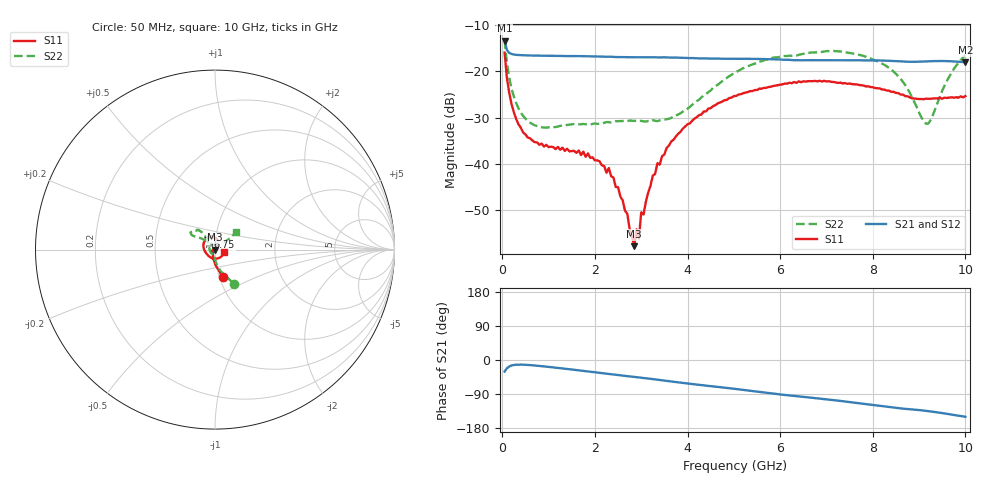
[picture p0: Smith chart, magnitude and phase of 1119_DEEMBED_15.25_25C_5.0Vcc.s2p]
!Hittite Microwave Corp.
!Digital Attenuator/PhaseShifter Rev 1.4.0
!Filename: C:\DATA\DATA\1119_DEEMBED_15.25_25C_5.0Vcc.s2p
!VNA ID: Agilent Technologies,N5224A,MY51441122,A.10.45.03
!Device type:
!2 Port Calibration.
!Temp(C): 25
!Lot Number:
!Serial Number:
!Operator:
!Misc:
!Attenuator:  15.250
# GHZ S DB R 50.0
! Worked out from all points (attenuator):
!   200 points, 50 MHz to 10 GHz, reference 50 ohm
!   highest |S21| = -13.29 dB at 50 MHz (marker M1); lowest = -18.0 dB at 10 GHz (marker M2)
!   lowest |S11| = -57.9 dB at 2.85 GHz (marker M3), VSWR 1.00, Z = 50 - j0.128 ohm
!   |S11| at or under -10 dB: start of sweep to end of sweep
!   |S22| runs from -32.2 to -13.3 dB; largest |S21 - S12| = 0.00049
!   S11 on the Smith chart (normalised r, x): 50 MHz: 1.04, -0.33; 6.75 GHz: 0.92, +0.13; 10 GHz: 1.11, -0.03
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0.05  -15.92 -74.2  -13.29 -30.4  -13.30 -30.5  -13.28 -61.1
0.1  -21.43 -88.5  -15.38 -21.8  -15.38 -21.8  -18.20 -75.7
0.2  -27.09 -102.7  -16.21 -14.5  -16.22 -14.5  -23.71 -87.1
0.45  -33.23 -125.1  -16.49 -12.3  -16.50 -12.4  -29.63 -97.7
0.85  -35.65 -147.3  -16.58 -16.2  -16.58 -16.2  -32.10 -106.0
1.75  -37.39 -159.4  -16.69 -28.8  -16.69 -28.8  -31.39 -116.4
2.3  -40.94 -162.7  -16.80 -37.0  -16.80 -37.0  -31.00 -131.7
2.7  -50.87 -115.3  -16.91 -42.6  -16.92 -42.7  -30.76 -142.3
2.85  -57.88 -89.0  -16.92 -44.8  -16.93 -44.8  -30.74 -148.8
2.9  -54.24 -22.4  -16.94 -45.3  -16.95 -45.4  -30.63 -151.3
2.95  -56.23 -49.8  -16.92 -46.0  -16.93 -46.0  -30.70 -153.7
3  -50.55 5.6  -16.92 -46.8  -16.93 -46.9  -30.72 -156.4
3.05  -51.02 6.9  -16.93 -47.6  -16.94 -47.6  -30.81 -158.5
3.4  -40.21 43.4  -16.94 -52.7  -16.95 -52.8  -30.62 -176.6
4  -31.43 52.4  -17.10 -61.9  -17.11 -62.0  -28.08 149.5
5.05  -25.30 73.1  -17.25 -76.6  -17.27 -76.6  -20.12 125.5
6.7  -22.12 118.5  -17.55 -99.8  -17.57 -99.8  -15.88 139.8
6.75  -22.04 119.2  -17.56 -100.5  -17.57 -100.5  -15.86 140.3
8.35  -24.16 176.9  -17.69 -123.9  -17.69 -123.9  -19.22 142.8
9.2  -25.92 -112.0  -17.80 -134.9  -17.81 -134.9  -31.29 82.0
9.6  -25.75 -66.2  -17.76 -142.1  -17.78 -142.1  -22.06 38.2
10  -25.33 -16.2  -18.02 -149.9  -18.02 -149.8  -16.44 39.7
